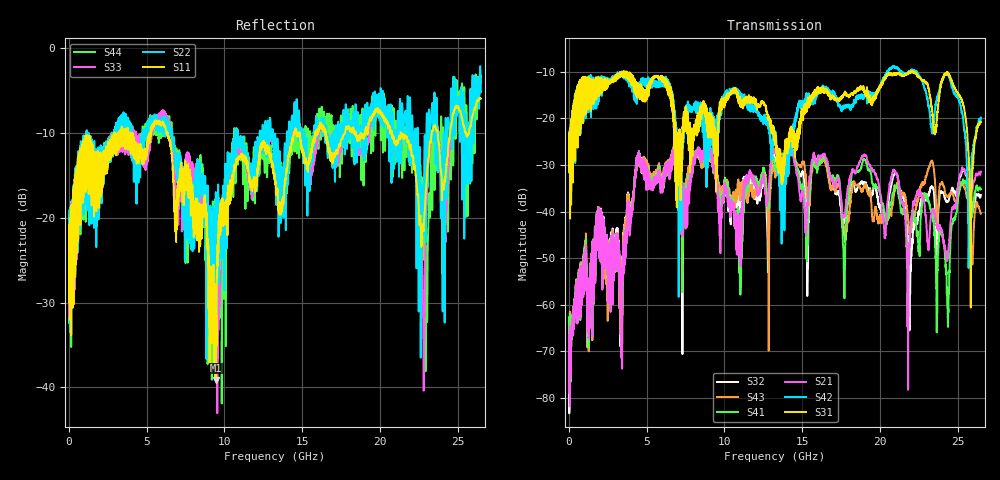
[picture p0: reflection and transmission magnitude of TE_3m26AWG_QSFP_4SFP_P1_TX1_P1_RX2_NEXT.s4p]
!Agilent Technologies,N5222A,MY51421691,A.10.00.00
!Agilent N5222A: A.10.00.00
!Date: Friday, January 30, 2015 12:34:08
!Correction: S11(Full 4 Port(1,2,3,4))
!S12(Full 4 Port(1,2,3,4))
!S13(Full 4 Port(1,2,3,4))
!S14(Full 4 Port(1,2,3,4))
!S21(Full 4 Port(1,2,3,4))
!S22(Full 4 Port(1,2,3,4))
!S23(Full 4 Port(1,2,3,4))
!S24(Full 4 Port(1,2,3,4))
!S31(Full 4 Port(1,2,3,4))
!S32(Full 4 Port(1,2,3,4))
!S33(Full 4 Port(1,2,3,4))
!S34(Full 4 Port(1,2,3,4))
!S41(Full 4 Port(1,2,3,4))
!S42(Full 4 Port(1,2,3,4))
!S43(Full 4 Port(1,2,3,4))
!S44(Full 4 Port(1,2,3,4))
!S4P File: Measurements: <S11,S12,S13,S14>,
!<S21,S22,S23,S24>,
!<S31,S32,S33,S34>,
!<S41,S42,S43,S44>:
# Hz S  dB  R 50.0
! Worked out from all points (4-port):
!   2650 points, 10 MHz to 26.5 GHz, reference 50 ohm
!   strongest paths, dB at 10 MHz, 6.63 GHz, 13.26 GHz, 19.88 GHz, 26.5 GHz:
!     S31: -24.8, -18.2, -24.4, -13.7, -20.8
!     S42: -24.7, -16.1, -25.0, -13.9, -19.9
!     S21: -66.5, -28.6, -26.9, -33.4, -31.5
!     S41: -62.7, -28.9, -30.1, -35.1, -35.2
!     S43: -71.8, -28.1, -31.9, -42.4, -40.4
!     S32: -66.1, -28.3, -28.5, -37.6, -36.5
!   lowest |S11| = -39.1 dB at 9.43 GHz (marker M1), VSWR 1.02, Z = 50.4 + j1.02 ohm
!   |S11| at or under -10 dB: start of sweep to 2.939 GHz; 6.342 GHz to 14.45 GHz (8.112 GHz wide, 78 % of centre); 21.36 GHz to 23.34 GHz (1.983 GHz wide, 8.87 % of centre)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
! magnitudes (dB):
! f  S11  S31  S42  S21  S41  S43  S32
! 10 MHz  -20.9  -24.8  -24.7  -66.5  -62.7  -71.8  -66.1
! 4.44 GHz  -12.3  -15.4  -14.9  -29.8  -30.0  -30.1  -29.8
! 9.43 GHz  -39.1  -27.5  -22.8  -32.1  -32.5  -32.7  -32.2
! 19.03 GHz  -10.1  -14.7  -15.4  -28.0  -28.9  -34.4  -33.9
! 24.36 GHz  -12.8  -10.4  -10.7  -49.4  -61.0  -36.9  -37.8
! 25.73 GHz  -10.0  -29.5  -47.7  -33.8  -36.3  -39.6  -33.9
! 26.5 GHz  -6.0  -20.8  -19.9  -31.5  -35.2  -40.4  -36.5
